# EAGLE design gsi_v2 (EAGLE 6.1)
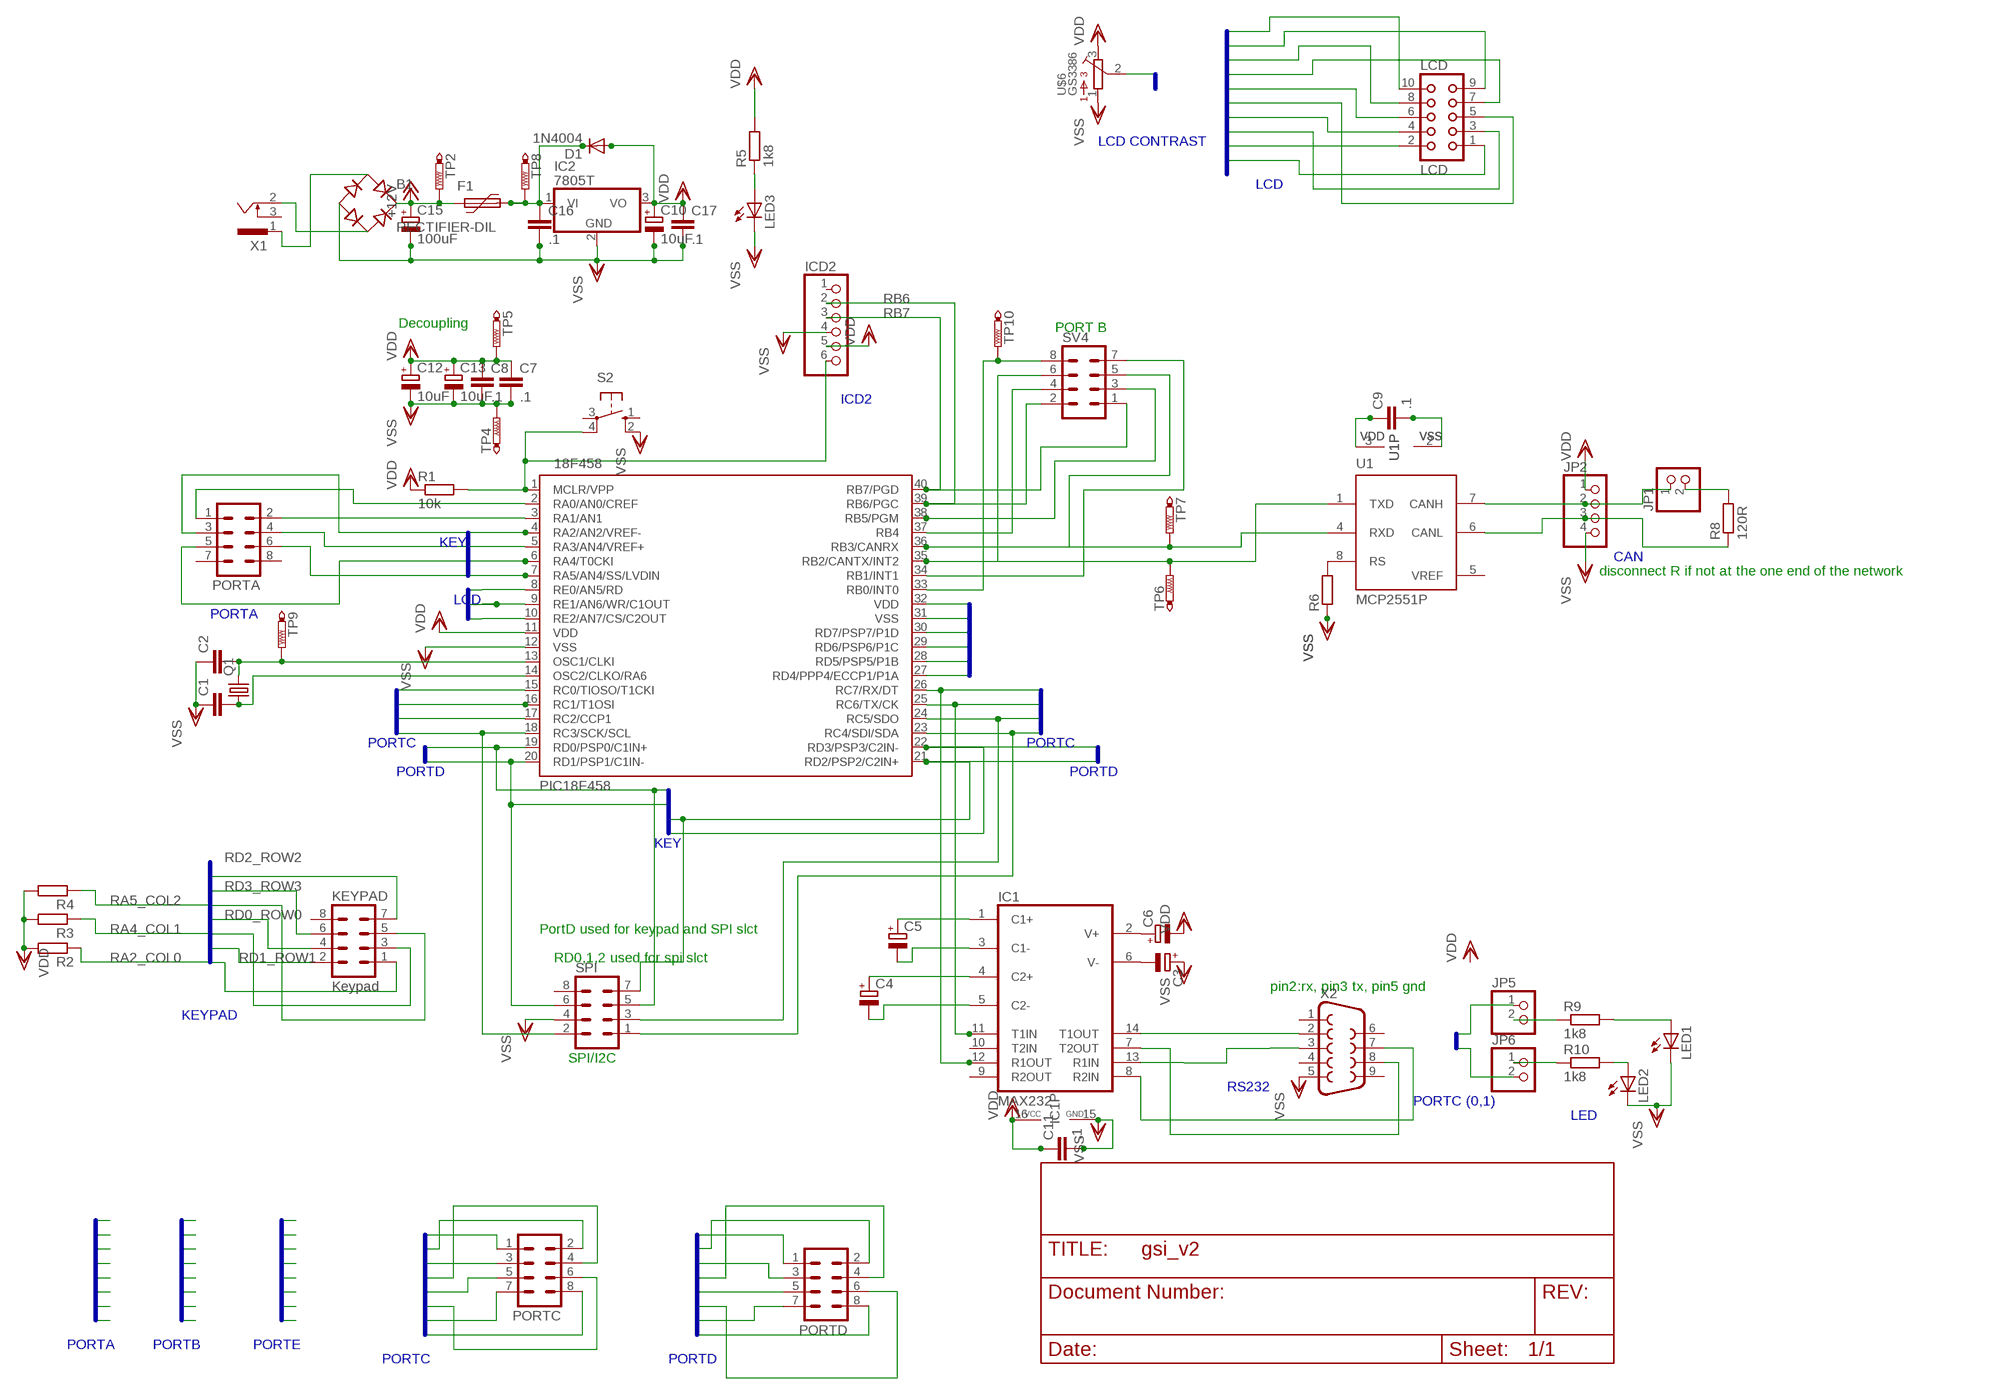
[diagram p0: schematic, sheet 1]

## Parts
B1  RECTIFIER-DIL  [B-DIL]
C1  C-EUC0603  [C0603]
C2  C-EUC0603  [C0603]
C3  CPOL-EUE2.5-6  [E2,5-6]
C4  CPOL-EUE2.5-6  [E2,5-6]
C5  CPOL-EUE2.5-6  [E2,5-6]
C6  CPOL-EUE2.5-6  [E2,5-6]
C7  .1  C-EUC0603  [C0603]
C8  .1  C-EUC0603  [C0603]
C9  .1  C-EUC0603  [C0603]
C10  10uF  CPOL-EUE2.5-5  [E2,5-5]
C11  .1  C-EUC0603  [C0603]
C12  10uF  CPOL-EUE2.5-5  [E2,5-5]
C13  10uF  CPOL-EUE2.5-5  [E2,5-5]
C15  100uF  CPOL-EUE2.5-7  [E2,5-7]
C16  .1  C-EUC0603  [C0603]
C17  .1  C-EUC0603  [C0603]
D1  1N4004  [DO41-10]
F1  MF-R055-5,1  [MF-5,1]
IC1  MAX232  [DIL16]
IC2  7805T  [TO220H]
ICD2  PINHD-1X6  [1X06]
JP1  PINHD-1X2  [1X02]
JP2  PINHD-1X4  [1X04]
JP5  PINHD-1X2  [1X02]
JP6  PINHD-1X2  [1X02]
KEYPAD  Keypad  MA04-2  [MA04-2]
LCD  LCD  CON10  [CON10]
LED1  LED5MM  [LED5MM]
LED2  LED5MM  [LED5MM]
LED3  LEDCHIPLED_1206  [CHIPLED_1206]
PORTA  MA04-2  [MA04-2]
PORTC  MA04-2  [MA04-2]
PORTD  MA04-2  [MA04-2]
Q1  CRYSTALHC18U-V  [HC18U-V]
R1  10k  R-EU_R0603  [R0603]
R2  R-EU_R0603  [R0603]
R3  R-EU_R0603  [R0603]
R4  R-EU_R0603  [R0603]
R5  1k8  R-EU_R0603  [R0603]
R6  R-EU_R0603  [R0603]
R8  120R  R-EU_0204/2V  [0204V]
R9  1k8  R-EU_R0603  [R0603]
R10  1k8  R-EU_R0603  [R0603]
S2  10-XX  [B3F-10XX]
SPI  MA04-2  [MA04-2]
SV4  MA04-2  [MA04-2]
TP2  PTR1PAD1-17  [P1-17]
TP4  PTR1PAD1-17  [P1-17]
TP5  PTR1PAD1-17  [P1-17]
TP6  PTR1PAD1-17  [P1-17]
TP7  PTR1PAD1-17  [P1-17]
TP8  PTR1PAD1-17  [P1-17]
TP9  PTR1PAD1-17  [P1-17]
TP10  PTR1PAD1-17  [P1-17]
U1  MCP2551P  [DIL8]
U$1  PIC18F458  [DIL40]
U$6  GS3386  [GS3386W]
X1  SCD-014A  [SCD-014-A]
X2  F09HP  [F09HP]

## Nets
+12V [power]: B1.+ C15.+ F1.1 TP2.1(TP)
C1+: C5.+ IC1.1(C1+)
C1-: C5.- IC1.3(C1-)
C2+: C4.+ IC1.4(C2+)
C2-: C4.- IC1.5(C2-)
CAN [power]: JP2.4 ; supply symbol labelled VSS
CANH: JP1.1 JP2.2 U1.7(CANH)
CANL: JP2.3 R8.1 U1.6(CANL)
CTS: IC1.7(T2OUT) X2.8
D4: LCD.10 U$1.27(RD4/PPP4/ECCP1/P1A)
D5: LCD.9 U$1.28(RD5/PSP5/P1B)
D6: LCD.8 U$1.29(RD6/PSP6/P1C)
D7: LCD.7 U$1.30(RD7/PSP7/P1D)
EN: LCD.1 U$1.8(RE0/AN5/RD)
LED1: LED1.A R9.2
LED2: LED2.A R10.2
MCLR: ICD2.6 R1.2 S2.4(P1) U$1.1(MCLR/VPP)
N$2: C2.2 Q1.2 TP9.1(TP) U$1.13(OSC1/CLKI)
N$3 [power]: B1.AC2 X1.2
N$4: C3.- IC1.6(V-)
N$5: C6.+ IC1.2(V+)
N$6: C1.2 Q1.1 U$1.14(OSC2/CLKO/RA6)
N$8: R6.2 U1.8(RS)
N$9 [power]: B1.AC1 X1.1
N$10 [power]: C16.1 D1.C F1.2 IC2.1(VI) TP8.1(TP)
N$13: JP6.1 R10.1
N$16: JP1.2 R8.2
N$17: JP5.2 R9.1
N$18: LED3.A R5.1
RA0: PORTA.1 U$1.2(RA0/AN0/CREF)
RA1: PORTA.2 U$1.3(RA1/AN1)
RA2_COL0: KEYPAD.1 PORTA.3 R2.1 U$1.4(RA2/AN2/VREF-)
RA3: PORTA.4 U$1.5(RA3/AN4/VREF+)
RA4_COL1: KEYPAD.3 PORTA.5 R3.1 U$1.6(RA4/T0CKI)
RA5_COL2: KEYPAD.5 PORTA.6 R4.1 U$1.7(RA5/AN4/SS/LVDIN)
RB0: SV4.8 TP10.1(TP) U$1.33(RB0/INT0)
RB1: SV4.7 U$1.34(RB1/INT1)
RB2: SV4.6 TP6.1(TP) U1.1(TXD) U$1.35(RB2/CANTX/INT2)
RB3: SV4.5 TP7.1(TP) U1.4(RXD) U$1.36(RB3/CANRX)
RB4: SV4.4 U$1.37(RB4)
RB5: SV4.3 U$1.38(RB5/PGM)
RB6: ICD2.2 SV4.2 U$1.39(RB6/PGC)
RB7: ICD2.3 SV4.1 U$1.40(RB7/PGD)
RC0: JP5.1 PORTC.1 U$1.15(RC0/TIOSO/T1CKI)
RC1: JP6.2 PORTC.2 U$1.16(RC1/T1OSI)
RC2: PORTC.3 U$1.17(RC2/CCP1)
RC3: PORTC.4 SPI.2 U$1.18(RC3/SCK/SCL)
RC4: PORTC.5 SPI.1 U$1.23(RC4/SDI/SDA)
RC5: PORTC.6 SPI.3 U$1.24(RC5/SDO)
RC6: IC1.11(T1IN) PORTC.7 U$1.25(RC6/TX/CK)
RC7: IC1.12(R1OUT) PORTC.8 U$1.26(RC7/RX/DT)
RD0_ROW0: KEYPAD.4 PORTD.1 SPI.5 U$1.19(RD0/PSP0/C1IN+)
RD1_ROW1: KEYPAD.2 PORTD.2 SPI.6 U$1.20(RD1/PSP1/C1IN-)
RD2_ROW2: KEYPAD.7 PORTD.3 SPI.7 U$1.21(RD2/PSP2/C2IN+)
RD3_ROW3: KEYPAD.6 PORTD.4 U$1.22(RD3/PSP3/C2IN-)
RD4: PORTD.5
RD5: PORTD.6
RD6: PORTD.7
RD7: PORTD.8
RS: LCD.3 U$1.10(RE2/AN7/CS/C2OUT)
RTS: IC1.8(R2IN) X2.7
RW: LCD.2 U$1.9(RE1/AN6/WR/C1OUT)
RX_232: IC1.13(R1IN) X2.3
TX_232: IC1.14(T1OUT) X2.2
VDD [power]: C6.- C7.1 C8.1 C9.1 C10.+ C11.1 C12.+ C13.+ C17.1 D1.A IC1.16(VCC) IC2.3(VO) ICD2.5 JP2.1 LCD.4 R1.1 R2.2 R3.2 R4.2 R5.2 TP5.1(TP) U1.3(VDD) U$1.11(VDD) U$1.32(VDD) U$6.3
VO: LCD.6 U$6.2
VSS [power]: B1.- C1.1 C2.1 C3.+ C7.2 C8.2 C9.2 C10.- C11.2 C12.- C13.- C15.- C16.2 C17.2 IC1.15(GND) IC2.2(GND) ICD2.4 LCD.5 LED1.K(C) LED2.K(C) LED3.C R6.1 S2.2(S1) SPI.4 TP4.1(TP) U1.2(VSS) U$1.12(VSS) U$1.31(VSS) U$6.1 X2.5
Unconnected: IC1.9(R2OUT) IC1.10(T2IN) ICD2.1 KEYPAD.8 PORTA.7 PORTA.8 S2.1(S) S2.3(P) SPI.8 X1.3 X2.1 X2.4 X2.6 X2.9

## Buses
LCD_BUS
KEYPAD_BUS
PORTD
PORTC
PORTE
PORTB
PORTA
VDD,VSS,RS,VO,EN,RW,D4,D5,D6,D7

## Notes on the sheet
- LCD CONTRAST
- LCD
- Decoupling
- PORT B
- ICD2
- KEY
- CAN
- disconnect R if not at the one end of the network
- LCD
- PORTA
- PORTC | PORTC
- PORTD | PORTD
- KEY
- PortD used for keypad and SPI slct
- RD0,1,2 used for spi slct
- pin2:rx, pin3 tx, pin5 gnd
- KEYPAD
- SPI/I2C
- RS232
- PORTC (0,1)
- LED
- PORTA | PORTB | PORTE
- PORTC | PORTD

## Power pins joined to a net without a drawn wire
VREF: U1.5(VREF)

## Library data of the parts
B1 = rectifier:RECTIFIER-: Rectifier
C1 C2 C7-C9 C11 C16 C17 = rcl:C-EU: CAPACITOR, European symbol
C3-C6 C10 C12 C13 C15 = rcl:CPOL-EU: POLARIZED CAPACITOR, European symbol
D1 = diode:1N4004: DIODE
F1 = bourns:MF-R055: MultiFuse
IC1 = maxim:MAX232: RS232 TRANSEIVER
IC2 = linear:78*: Positive VOLTAGE REGULATOR Source: http://cache.national.com/ds/LM/LM78L05.pdf http://www.fairchildsemi.com/ds/LM/LM7805.pdf
ICD2 = pinhead:PINHD-1X6: PIN HEADER
JP1 JP5 JP6 = pinhead:PINHD-1X2: PIN HEADER
JP2 = pinhead:PINHD-1X4: PIN HEADER
KEYPAD PORTA PORTC PORTD SPI SV4 = con-lstb:MA04-2: PIN HEADER
LCD = con-harting:CON10: CONNECTOR; OC_FARNELL: unknown; OC_NEWARK: unknown
LED1-LED3 = led:LED: LED
Q1 = crystal:CRYSTAL: CRYSTAL
R1-R6 R8-R10 = rcl:R-EU_: RESISTOR, European symbol
S2 = switch-omron:10-XX: OMRON SWITCH
TP2 TP4-TP10 = testpad:PTR1: TEST PIN
U1 = microchip_can:MCP2551: High Speed CAN tranceiver
U$1 = gs:PIC18F458
U$6 = gs:GS3386: GS larger pads
X1 = con-shiua-chyuan:SCD-014A: Power Jack 2.5mm
X2 = con-subd:F09: SUB-D

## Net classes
0 default: width 0.457 mm, drill 0.813 mm, clearance 0.254 mm
1 power: width 1.016 mm, drill 0.813 mm, clearance 0.508 mm
2 digital: width 0.457 mm, drill 0.813 mm, clearance 0.254 mm

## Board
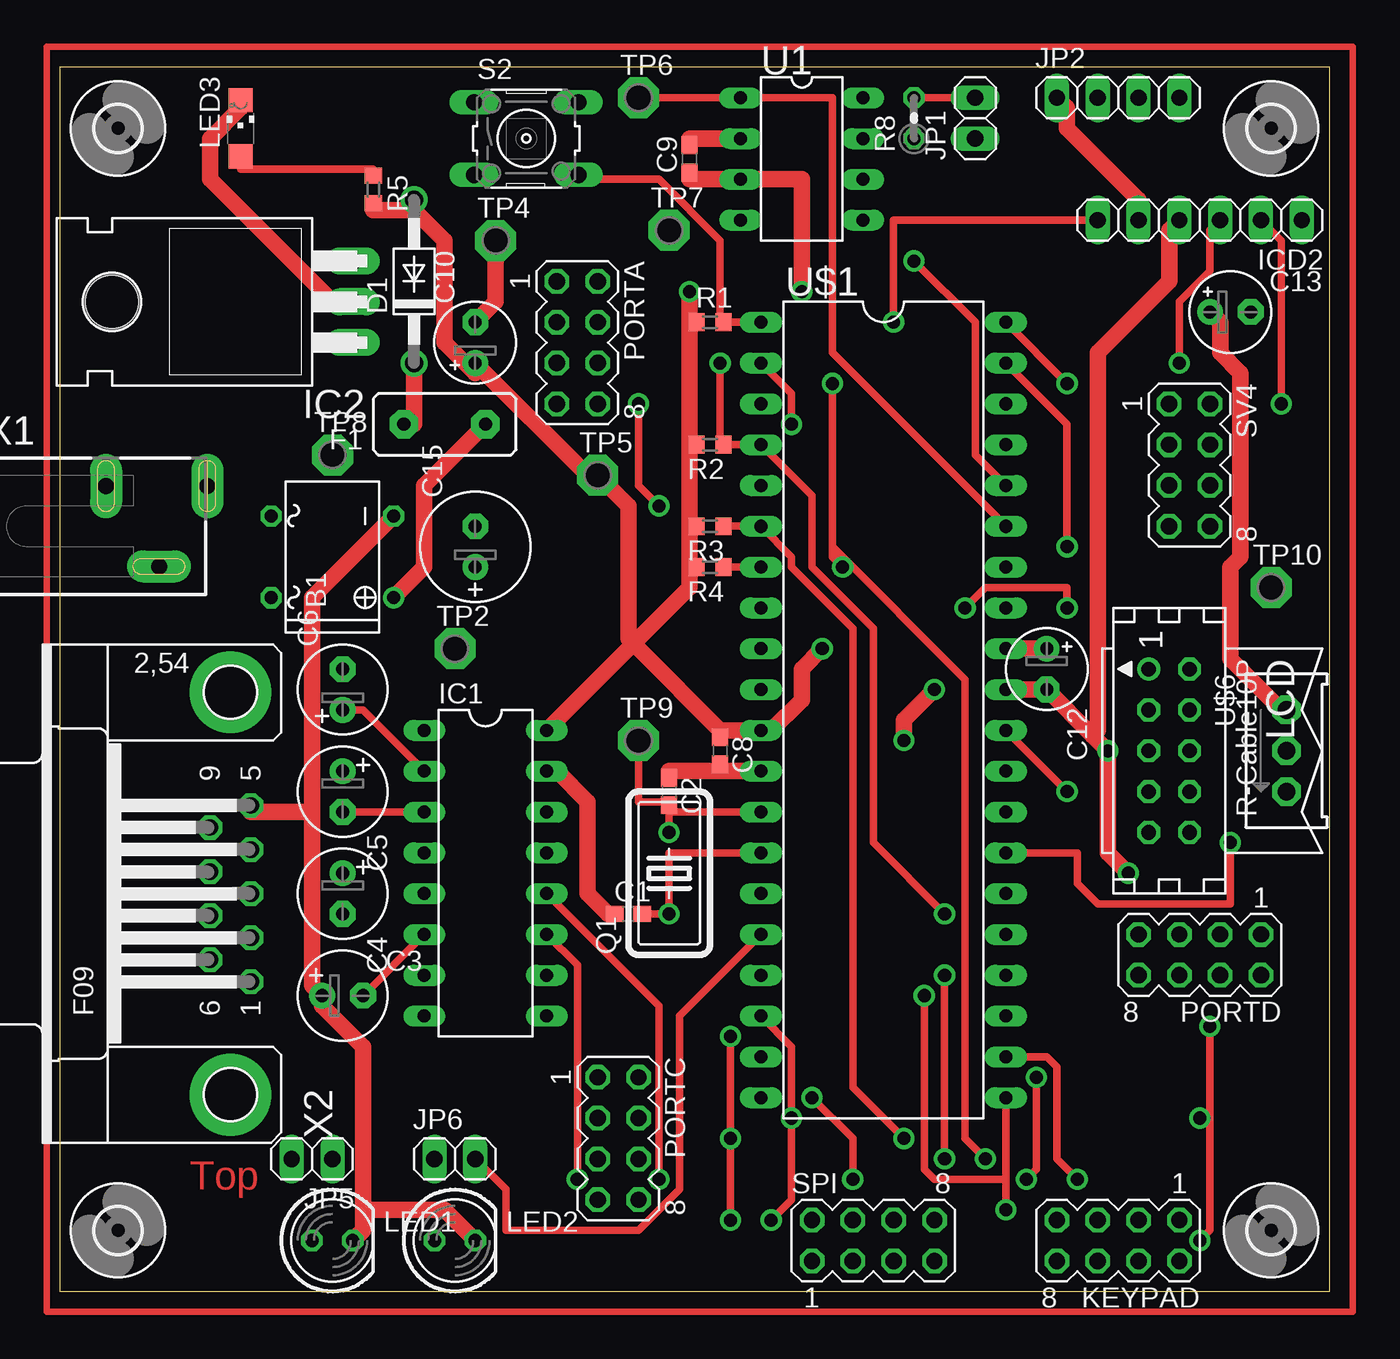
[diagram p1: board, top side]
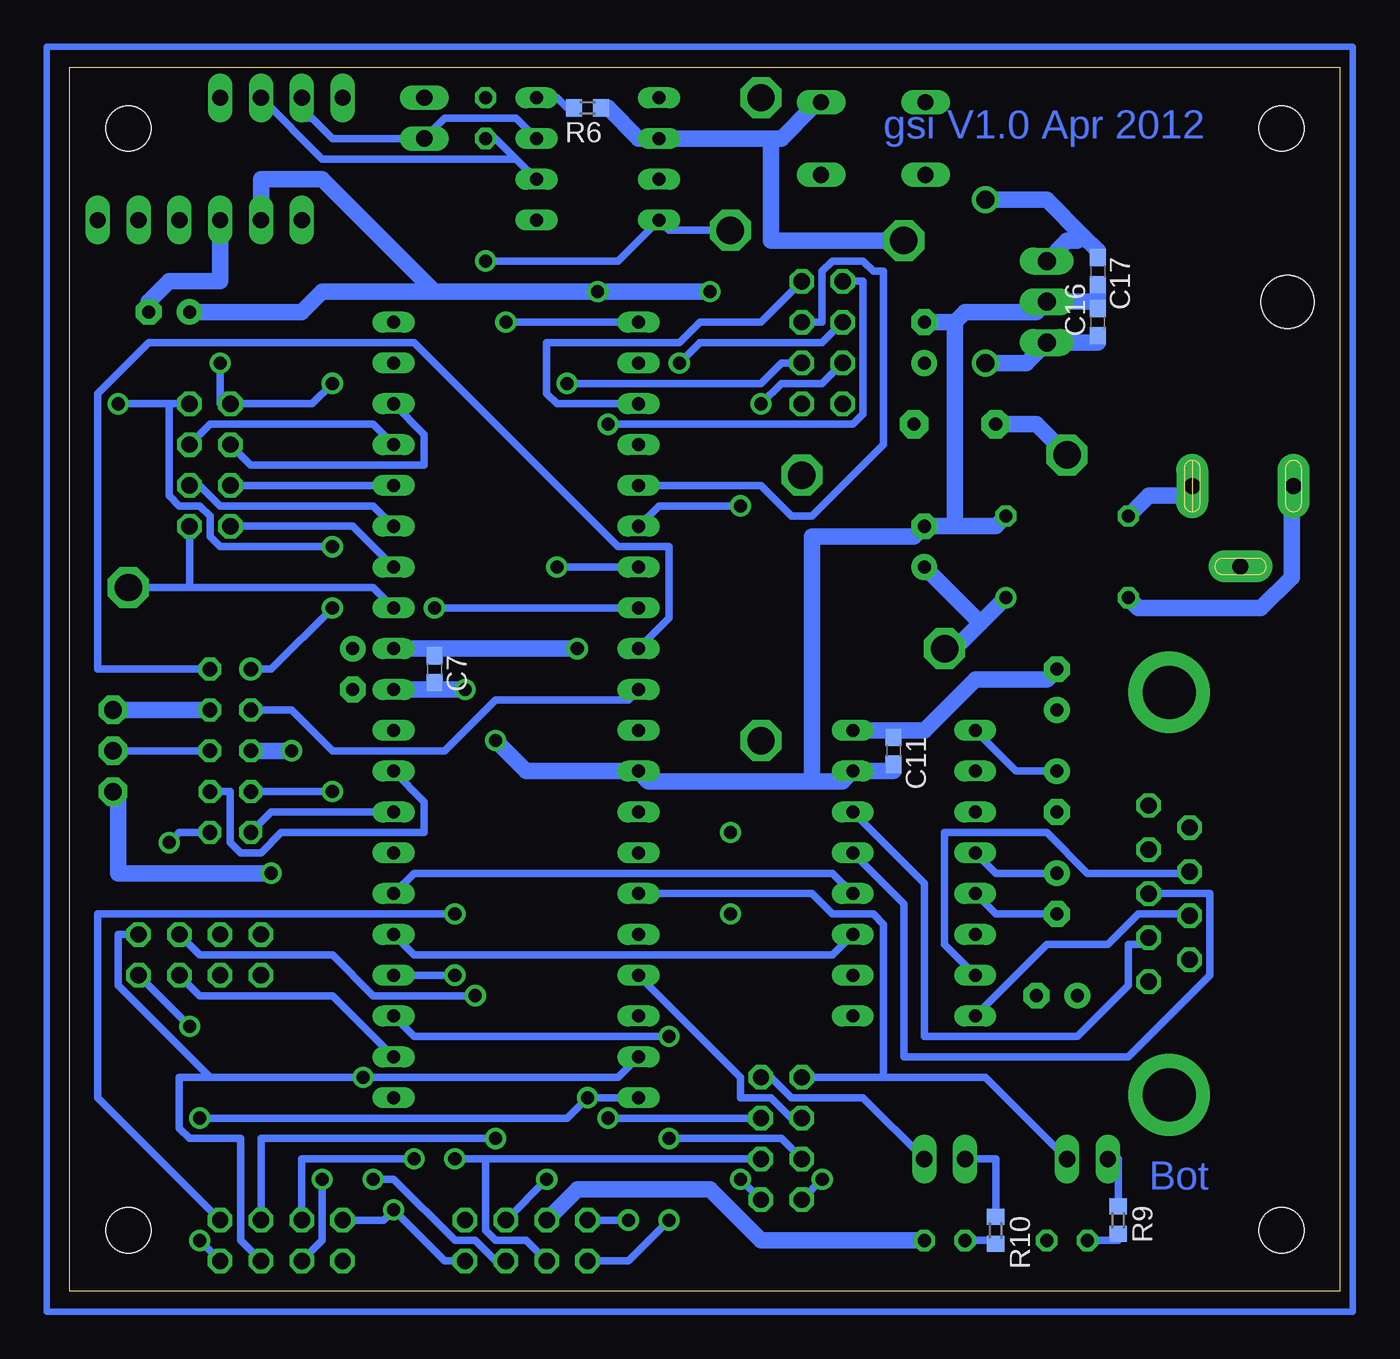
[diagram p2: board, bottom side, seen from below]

Size 79.05 x 76.19 mm. Coordinates in mm from the lower left corner, seen from the top.
Outline: 0,0 79.05,0 79.05,76.19 0,76.19 0,0
Copper layers (1*16): Top 0.035mm / dielectric 1.5mm / Bottom 0.035mm
Design rules: minimum track width 10mil, minimum drill 24mil, track to track 10mil, track to pad 10mil, pad to pad 10mil, via to via 10mil, smd to smd 10mil, copper to edge 40mil, drill to drill 10mil, minimum pad ring 10mil, minimum via ring 10mil, stop-mask expansion 4mil, vias tented up to drill 0mil, thermal gap 10mil
tRestrict: area 33.5,4.4 to 36,14.6; area 45.6,1.9 to 55.7,4.4; area 26.5,69.8 to 31.6,74.9; area 67.8,46.4 to 72.9,56.5; area 65.9,18.4 to 76,23.5; area 66.5,27.3 to 71.6,41.3; area 60.8,1.9 to 69.7,5.1; area 30.3,54.6 to 34.1,63.5

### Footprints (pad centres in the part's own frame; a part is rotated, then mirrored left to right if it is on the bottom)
B-DIL = drill 0.813: + -2.54,-3.81 | drill 0.813 octagon: - 2.54,-3.81; AC1 2.54,3.81; AC2 -2.54,3.81
C0603 = smd 1.1 x 1: 1 -0.85,0; 2 0.85,0
E2,5-6 = drill 0.813 pad 1.6: + -1.27,0 | drill 0.813 pad 1.6 octagon: - 1.27,0
E2,5-5 = drill 0.813 pad 1.6: + -1.27,0 | drill 0.813 pad 1.6 octagon: - 1.27,0
E2,5-7 = drill 0.813 pad 1.6: + -1.27,0 | drill 0.813 pad 1.6 octagon: - 1.27,0
DO41-10 = drill 1.118: A 5.08,0; C -5.08,0
MF-5,1 = drill 0.813 pad 1.778 octagon: 1 -2.54,0; 2 2.54,0
DIL16 = drill 0.813 long: 1 -8.89,-3.81; 2 -6.35,-3.81; 3 -3.81,-3.81; 4 -1.27,-3.81; 5 1.27,-3.81; 6 3.81,-3.81; 7 6.35,-3.81; 8 8.89,-3.81; 9 8.89,3.81; 10 6.35,3.81; 11 3.81,3.81; 12 1.27,3.81; 13 -1.27,3.81; 14 -3.81,3.81; 15 -6.35,3.81; 16 -8.89,3.81
TO220H = drill 1.118 long: 1 -2.54,-10.16; 2 0,-10.16; 3 2.54,-10.16 | hole 3.302: 0,4.826
1X06 = drill 1.016 long: 1 -6.35,0; 2 -3.81,0; 3 -1.27,0; 4 1.27,0; 5 3.81,0; 6 6.35,0
1X02 = drill 1.016 long: 1 -1.27,0; 2 1.27,0
1X04 = drill 1.016 long: 1 -3.81,0; 2 -1.27,0; 3 1.27,0; 4 3.81,0
MA04-2 = drill 1.016 octagon: 1 -3.81,-1.27; 2 -3.81,1.27; 3 -1.27,-1.27; 4 -1.27,1.27; 5 1.27,-1.27; 6 1.27,1.27; 7 3.81,-1.27; 8 3.81,1.27
CON10 = drill 0.914: 1 -5.08,-1.27 | drill 0.914 octagon: 2 -5.08,1.27; 3 -2.54,-1.27; 4 -2.54,1.27; 5 0,-1.27; 6 0,1.27; 7 2.54,-1.27; 8 2.54,1.27; 9 5.08,-1.27; 10 5.08,1.27
LED5MM = drill 0.813 octagon: A -1.27,0; K 1.27,0
CHIPLED_1206 = smd 1.5 x 1.5: A 0,-1.75; C 0,1.75
HC18U-V = drill 0.813: 1 -2.54,0; 2 2.54,0
R0603 = smd 1 x 1.1: 1 -0.85,0; 2 0.85,0
0204V = drill 0.813 octagon: 1 -1.27,0; 2 1.27,0
B3F-10XX = drill 1.016 long: 1 -3.251,2.261; 2 3.251,2.261; 3 -3.251,-2.261; 4 3.251,-2.261
P1-17 = drill 1.702 pad 2.54 octagon: 1 0,0
DIL8 = drill 0.813 long: 1 -3.81,-3.81; 2 -1.27,-3.81; 3 1.27,-3.81; 4 3.81,-3.81; 5 3.81,3.81; 6 1.27,3.81; 7 -1.27,3.81; 8 -3.81,3.81
DIL40 = drill 0.813 long: 1 -24.13,-7.62; 2 -21.59,-7.62; 3 -19.05,-7.62; 4 -16.51,-7.62; 5 -13.97,-7.62; 6 -11.43,-7.62; 7 -8.89,-7.62; 8 -6.35,-7.62; 9 -3.81,-7.62; 10 -1.27,-7.62; 11 1.27,-7.62; 12 3.81,-7.62; 13 6.35,-7.62; 14 8.89,-7.62; 15 11.43,-7.62; 16 13.97,-7.62; 17 16.51,-7.62; 18 19.05,-7.62; 19 21.59,-7.62; 20 24.13,-7.62; 21 24.13,7.62; 22 21.59,7.62; 23 19.05,7.62; 24 16.51,7.62; 25 13.97,7.62; 26 11.43,7.62; 27 8.89,7.62; 28 6.35,7.62; 29 3.81,7.62; 30 1.27,7.62; 31 -1.27,7.62; 32 -3.81,7.62; 33 -6.35,7.62; 34 -8.89,7.62; 35 -11.43,7.62; 36 -13.97,7.62; 37 -16.51,7.62; 38 -19.05,7.62; 39 -21.59,7.62; 40 -24.13,7.62
2,8 = hole 2.8: 0,0
GS3386W = drill 1.1 pad 1.778 octagon: 1 2.54,0.318; 2 0,0.318; 3 -2.54,0.318
SCD-014-A = drill 1 pad 2 long: 1 -2.5,13.8; 2 -2.5,7.5; 3 2.5,10.8
F09HP = drill 1.016 octagon: 1 -5.486,-1.27; 2 -2.743,-1.27; 3 0,-1.27; 4 2.743,-1.27; 5 5.486,-1.27; 6 -4.115,1.27; 7 -1.372,1.27; 8 1.372,1.27; 9 4.115,1.27 | drill 3.302 pad 5.08: G1 -12.522,0; G2 12.522,0

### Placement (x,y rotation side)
B1  16.98,45.71 90 top
C1  35.39,23.49 0 top
C2  37.94,31.11 270 top
C3  17.61,18.41 0 top
C4  17.61,24.76 270 top
C5  17.61,31.11 270 top
C6  17.61,37.46 90 top
C7  56.35,38.73 270 bottom
C8  41.11,33.65 270 top
C9  39.2,70.48 90 top
C10  25.87,59.05 90 top
C11  27.78,33.65 270 bottom
C12  61.43,38.73 270 top
C13  72.86,60.95 0 top
C15  25.87,46.35 90 top
C16  15.07,60.32 90 bottom
C17  15.07,63.5 270 bottom
D1  22.06,62.86 90 top
F1  23.96,53.97 180 top
IC1  26.5,26.03 270 top
IC2  8.09,61.59 90 top
ICD2  70.95,66.67 180 top
JP1  56.98,73.02 90 top
JP2  65.88,74.29 0 top
JP5  15.71,8.25 180 top
JP6  24.6,8.25 0 top
KEYPAD  65.88,3.17 180 top
LCD  69.05,33.65 270 top
LED1  16.98,3.17 0 top
LED2  24.6,3.17 0 top
LED3  11.26,72.39 0 top
PORTA  32.22,59.05 270 top
PORTC  34.76,9.52 270 top
PORTD  70.95,20.95 180 top
Q1  37.94,26.03 90 top
R1  40.47,60.32 0 top
R2  40.47,52.7 180 top
R3  40.47,47.62 180 top
R4  40.47,45.08 180 top
R5  19.52,68.58 270 top
R6  46.82,73.66 180 bottom
R8  53.17,73.02 90 top
R9  13.8,4.44 270 bottom
R10  21.43,3.8 270 bottom
S2  29.04,71.75 0 top
SPI  50.63,3.17 0 top
SV4  70.32,51.43 270 top
TP2  24.6,40 0 top
TP4  27.14,65.4 0 top
TP5  33.49,50.8 0 top
TP6  36.03,74.29 0 top
TP7  37.94,66.03 0 top
TP8  16.98,52.06 0 top
TP9  36.03,34.28 0 top
TP10  75.4,43.81 0 top
U1  46.19,70.48 270 top
U$1  51.27,36.19 270 top
U$2  [2,8]  3.64,72.39 0 top
U$3  [2,8]  75.4,72.39 0 top
U$4  [2,8]  75.4,3.8 0 top
U$5  [2,8]  3.64,3.8 0 top
U$6  76.03,33.65 270 top
X1  -4.61,47.62 270 top
X2  10.63,24.76 90 top

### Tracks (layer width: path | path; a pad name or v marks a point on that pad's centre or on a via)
+12V
  Top 1.016: F1.1 22.69,50.16 22.69,45.08 B1.+
  Bottom 1.016: 22.38,41.59 23.96,40 TP2.1 | 22.38,41.59 B1.+ | C15.+ 22.69,41.91 22.38,41.59
C1+
  Bottom 0.457: IC1.1 20.15,32.38 C5.+
C1-
  Top 0.457: C5.- IC1.3
C2+
  Bottom 0.457: IC1.4 21.43,26.03 C4.+
C2-
  Bottom 0.457: IC1.5 21.43,23.49 C4.-
CANH
  Bottom 0.457: U1.7 51.27,73.02 55.71,73.02 JP1.1 62.7,71.75 63.97,73.02 64.6,73.02 JP2.2
CANL
  Bottom 0.457: 51.27,70.48 52.54,71.75 R8.1 | 51.27,70.48 U1.6 | JP2.3 63.33,70.48 51.27,70.48
CTS
  Bottom 0.457: IC1.7 24.6,21.59 24.6,28.57 18.25,28.57 15.71,26.03 9.36,26.03 X2.8
D4  (via drill 0.81)
  Top 0.457: U$1.27 63.33,27.3 63.33,25.4 64.6,24.12 72.86,24.12 v72.86,27.94
  Bottom 0.457: v72.86,27.94 72.22,28.57 LCD.10
D5
  Bottom 0.457: U$1.28 66.51,29.84 LCD.9
D6
  Bottom 0.457: U$1.29 56.98,30.48 56.98,28.57 65.88,28.57 67.14,27.3 68.41,27.3 69.05,27.94 69.05,31.11 LCD.8
D7  (via drill 0.81)
  Top 0.457: v62.7,31.11 U$1.30
  Bottom 0.457: LCD.7 v62.7,31.11
EN  (via drill 0.81)
  Top 0.457: v56.35,42.54 57.62,43.81 62.7,43.81 v62.7,42.54
  Bottom 0.457: v56.35,42.54 U$1.8 | v62.7,42.54 66.51,38.73 LCD.1
LED1
  Bottom 0.457: LED1.A 13.8,3.17 R9.2
LED2
  Bottom 0.457: LED2.A 21.43,3.17 R10.2
MCLR  (via drill 0.81)
  Top 0.457: U$1.1 41.75,60.32 R1.2 41.11,60.32 41.11,65.4 37.3,69.21 32.86,69.21 S2.4 | ICD2.6 51.91,66.67 v51.91,60.32
  Bottom 0.457: U$1.1 v51.91,60.32
N$1
  Top 0.406: -0.8,77.47 -0.8,-1.27 80.48,-1.27 80.48,77.47 -0.8,77.47
N$2
  Top 0.457: Q1.2 37.94,29.84 | 37.94,29.84 C2.2 | 37.94,29.84 U$1.13 | 37.94,29.84 C2.2 | TP9.1 36.03,30.48 37.94,30.48 C2.2
N$3
  Bottom 1.016: B1.AC2 12.54,42.54 4.91,42.54 3.01,44.45 3.01,49.52 X1.2
N$4
  Top 0.457: C3.- IC1.6
N$5
  Top 0.457: IC1.2 18.89,36.19 C6.+
N$6
  Top 0.457: C1.2 36.66,23.49 Q1.1 37.94,27.3 U$1.14
N$7
  Bottom 0.406: -0.8,77.47 80.48,77.47 80.48,-1.27 -0.8,-1.27 -0.8,77.47
N$8
  Bottom 0.457: U1.8 48.73,74.29 48.09,73.66 R6.2
N$9
  Bottom 1.016: B1.AC1 11.9,49.52 9.36,49.52 X1.1
N$10
  Top 1.016: D1.C 22.06,53.97 F1.2
  Bottom 1.016: C16.1 15.07,59.05 IC2.1 19.52,57.78 D1.C | TP8.1 18.89,53.97 F1.2 | F1.2
N$11  (via drill 0.6 pad 2.54)
  other vias: 3.64,72.39
N$12  (via drill 0.6 pad 2.54)
  other vias: 75.4,72.39
N$13
  Bottom 0.457: JP6.1 21.43,8.25 21.43,5.08 R10.1
N$14  (via drill 0.6 pad 2.54)
  other vias: 3.64,3.8
N$15  (via drill 0.6 pad 2.54)
  other vias: 75.4,3.8
N$16
  Top 0.457: JP1.2 R8.2
N$17
  Bottom 0.457: JP5.2 13.8,8.25 13.8,5.71 R9.1
N$18
  Top 0.457: R5.1 19.52,69.84 11.26,69.84 11.26,70.48 LED3.A
RA0  (via drill 0.81)
  Top 0.457: U$1.2 45.55,55.88 v45.55,53.97
  Bottom 0.457: v45.55,53.97 30.32,53.97 29.68,54.6 29.68,62.86 PORTA.1
RA1
  Bottom 0.457: U$1.3 48.73,55.24 49.36,55.88 49.36,59.05 41.11,59.05 39.84,60.32 36.03,60.32 PORTA.2
RA2_COL0  (via drill 0.81)
  Top 0.457: v41.11,57.78 41.11,52.7 R2.1 41.75,52.7 U$1.4 46.82,49.52 46.82,45.08 50.63,41.27 50.63,27.94 v55.08,23.49
  Bottom 0.457: v41.11,57.78 39.84,59.05 32.22,59.05 PORTA.3 | KEYPAD.1 77.3,12.06 77.3,23.49 v55.08,23.49
RA3
  Bottom 0.457: U$1.5 36.03,50.16 34.12,48.25 32.86,48.25 28.41,52.7 28.41,63.5 29.04,63.5 29.68,64.13 31.58,64.13 32.22,63.5 32.22,60.32 PORTA.4
RA4_COL1  (via drill 0.81)
  Top 0.457: R3.1 41.75,47.62 U$1.6 45.55,45.71 45.55,45.08 49.36,41.27 49.36,12.7 v52.54,9.52 | v37.3,48.89 36.03,50.16 v36.03,55.24
  Bottom 0.457: U$1.6 42.38,48.89 v37.3,48.89 | v36.03,55.24 34.76,56.51 32.22,56.51 PORTA.5 | KEYPAD.3 67.14,9.52 v52.54,9.52
RA5_COL2  (via drill 0.81)
  Top 0.457: U$1.7 41.75,45.08 R4.1 | v48.73,45.08 48.09,45.71 48.09,46.35 | v48.09,56.51 48.09,46.35 | v57.62,8.25 56.35,9.52 56.35,38.09 48.09,46.35
  Bottom 0.457: v48.73,45.08 U$1.7 | v48.09,56.51 36.03,56.51 34.76,57.78 PORTA.6 | KEYPAD.5 64.6,8.25 v57.62,8.25
RB0
  Bottom 0.457: U$1.33 60.16,43.81 71.59,43.81 | TP10.1 71.59,43.81 | 71.59,43.81 SV4.8
RB1
  Bottom 0.457: U$1.34 61.43,47.62 SV4.7
RB2
  Top 0.457: TP6.1 U1.1 48.09,74.29 48.09,58.41 U$1.35
  Bottom 0.457: U$1.35 60.16,48.89 69.69,48.89 70.95,50.16 SV4.6
RB3  (via drill 0.81)
  Top 0.457: v53.17,64.13 56.98,60.32 56.98,52.06 U$1.36
  Bottom 0.457: TP7.1 41.75,66.03 U1.4 44.92,64.13 v53.17,64.13 | SV4.5 U$1.36
RB4
  Bottom 0.457: U$1.37 60.16,53.97 70.32,53.97 SV4.4
RB5
  Bottom 0.457: U$1.38 56.98,53.34 56.98,51.43 67.78,51.43 SV4.3
RB6  (via drill 0.81)
  Top 0.457: U$1.39 62.7,53.97 v62.7,46.35 | ICD2.2 76.03,65.4 v76.03,55.24
  Bottom 0.457: v62.7,46.35 69.69,46.35 70.32,46.98 70.32,48.25 70.95,48.89 72.22,48.89 72.86,49.52 72.86,55.24 | SV4.2 72.86,55.24 | 72.86,55.24 v76.03,55.24
RB7  (via drill 0.81)
  Top 0.457: v62.7,56.51 U$1.40 | ICD2.3 71.59,66.03 71.59,63.5 69.69,61.59 v69.69,57.78
  Bottom 0.457: v62.7,56.51 63.97,55.24 SV4.1 69.69,55.24 v69.69,57.78
RC0
  Bottom 0.457: U$1.15 32.86,24.76 31.58,23.49 29.04,23.49 28.41,22.85 28.41,13.33 | PORTC.1 28.41,13.33 | JP5.1 22.06,13.33 28.41,13.33
RC1
  Top 0.457: U$1.16 38.57,17.14 38.57,6.35 36.03,3.8 27.78,3.8 27.78,6.35 JP6.2
  Bottom 0.457: PORTC.2 35.39,13.33 34.12,12.06 29.68,12.06 JP6.2
RC2
  Bottom 0.457: U$1.17 37.3,13.33 37.3,12.06 35.39,12.06 34.12,10.79 PORTC.3
RC3  (via drill 0.81)
  Top 0.457: U$1.18 45.55,15.24 v45.55,10.79 45.55,5.71 v44.28,4.44
  Bottom 0.457: PORTC.4 v45.55,10.79 | v44.28,4.44 SPI.2
RC4  (via drill 0.81)
  Top 0.457: v41.75,4.44 v41.75,9.52 v41.75,15.87
  Bottom 0.457: U$1.23 57.62,15.87 v41.75,15.87 | v41.75,4.44 44.28,1.9 SPI.1 | PORTC.5 34.76,9.52 v41.75,9.52
RC5  (via drill 0.81)
  Top 0.457: v55.08,8.25 v55.08,19.68
  Bottom 0.457: v55.08,19.68 U$1.24 | PORTC.6 53.17,8.25 | 53.17,8.25 v55.08,8.25 | SPI.3 50.63,3.17 52.54,3.17 53.17,3.8 53.17,8.25
RC6  (via drill 0.81)
  Top 0.457: v32.22,6.98 32.22,20.31 IC1.11
  Bottom 0.457: IC1.11 31.58,20.95 57.62,20.95 U$1.25 | v32.22,6.98 PORTC.7
RC7  (via drill 0.81)
  Top 0.457: v37.3,6.98 37.3,17.77 IC1.12
  Bottom 0.457: IC1.12 31.58,26.03 57.62,26.03 U$1.26 | v37.3,6.98 PORTC.8
RD0_ROW0  (via drill 0.81)
  Top 0.457: v60.16,6.98 60.8,7.62 v60.8,13.33
  Bottom 0.457: U$1.19 44.92,13.33 v60.8,13.33 70.32,13.33 | 70.32,13.33 76.03,19.05 76.03,22.22 PORTD.1 | SPI.5 52.54,1.9 53.81,3.17 55.08,3.17 58.89,6.98 v60.16,6.98 | KEYPAD.4 68.41,3.17 68.41,9.52 71.59,9.52 72.22,10.15 72.22,13.33 70.32,13.33
RD1_ROW1  (via drill 0.81)
  Top 0.457: v46.82,12.06 49.36,9.52 v49.36,6.98 | v70.95,3.17 71.59,3.8 71.59,10.79 | v71.59,16.51 71.59,10.79 | 71.59,10.79 v70.95,10.79
  Bottom 0.457: U$1.20 v46.82,12.06 48.09,10.79 v70.95,10.79 | SPI.6 v49.36,6.98 | v70.95,3.17 KEYPAD.2 | PORTD.2 v71.59,16.51
RD2_ROW2  (via drill 0.81)
  Top 0.457: v58.89,5.08 58.89,6.98 | 58.89,6.98 U$1.21 | v53.81,18.41 53.81,7.62 54.44,6.98 58.89,6.98
  Bottom 0.457: KEYPAD.7 59.52,4.44 v58.89,5.08 55.71,1.9 SPI.7 | PORTD.3 70.95,20.95 62.7,20.95 60.16,18.41 v53.81,18.41
RD3_ROW3  (via drill 0.81)
  Top 0.457: v63.33,6.98 62.06,8.25 62.06,13.97 61.43,14.6 U$1.22
  Bottom 0.457: U$1.22 62.7,18.41 70.95,18.41 PORTD.4 | KEYPAD.6 63.33,3.17 v63.33,6.98
RS
  Bottom 0.457: U$1.10 44.28,36.82 52.54,36.82 55.71,33.65 62.7,33.65 65.24,36.19 LCD.3
RTS
  Bottom 0.457: IC1.8 18.25,21.59 14.44,21.59 12.54,23.49 9.36,23.49 X2.7
RW
  Bottom 0.457: U$1.9 41.75,41.91 41.75,46.35 44.92,46.35 57.62,59.05 74.13,59.05 77.3,55.88 77.3,38.73 LCD.2
RX_232
  Bottom 0.457: IC1.13 27.14,24.12 27.14,14.6 13.17,14.6 8.09,19.68 8.09,24.76 X2.3
TX_232
  Bottom 0.457: IC1.14 25.87,25.4 25.87,15.87 16.35,15.87 13.17,19.05 13.17,21.59 11.9,21.59 X2.2
VDD  (via drill 0.81)
  Top 1.016: JP2.1 62.7,73.66 62.7,72.39 67.14,67.94 ICD2.5 | C9.1 39.2,69.21 U1.3 46.19,69.21 v46.19,62.22 | C13.+ 72.22,60.32 72.22,58.41 73.49,57.14 73.49,45.71 72.86,45.08 72.86,39.36 76.03,36.19 U$6.3 | 22.06,67.3 19.52,67.3 R5.2 | 22.06,67.3 D1.A 22.06,67.3 | 22.06,67.3 23.96,65.4 23.96,59.05 25.87,57.14 C10.+ 32.86,50.8 TP5.1 35.39,48.89 35.39,40.63 35.71,40.32 | C12.+ U$1.32 | 41.11,34.92 U$1.11 44.28,34.92 46.19,36.82 46.19,38.73 v47.46,40 | 41.11,34.92 C8.1 41.11,34.92 | 39.2,47.62 39.2,45.08 | 39.2,45.08 R4.2 39.2,45.08 | 39.2,47.62 R3.2 39.2,47.62 | 39.2,47.62 39.2,52.7 | 39.2,52.7 R2.2 39.2,52.7 | 39.2,52.7 39.2,60.32 | 39.2,60.32 R1.1 39.2,60.32 | 35.71,40.32 39.2,43.81 39.2,45.08 | 35.71,40.32 IC1.16 | 41.11,34.92 36.03,40 35.71,40.32 | 39.2,60.32 v39.2,62.22
  Bottom 1.016: LCD.4 76.03,36.19 U$6.3 | 56.35,62.22 63.33,62.22 64.6,60.95 C13.+ | 56.35,62.22 v46.19,62.22 v39.2,62.22 | ICD2.5 67.14,69.21 63.33,69.21 56.35,62.22 | 16.03,65.72 18.25,67.94 D1.A | 16.03,65.72 15.07,64.77 C17.1 | IC2.3 16.98,65.4 16.35,65.4 16.03,65.72 | U$1.32 56.35,40 | 56.35,40 C7.1 56.35,40 | IC1.16 27.78,34.92 | 27.78,34.92 C11.1 27.78,34.92 | C6.- 18.25,38.09 22.69,38.09 25.87,34.92 27.78,34.92 | v47.46,40 56.35,40
VO
  Bottom 0.457: LCD.6 76.03,33.65 U$6.2
VSS  (via drill 0.81)
  Top 1.016: LED1.K 18.89,3.8 18.89,5.08 | 18.89,5.08 18.89,15.24 16.35,17.77 C3.+ 15.71,19.05 15.71,29.84 | LED2.K 23.96,5.08 18.89,5.08 | 15.71,29.84 11.9,29.84 X2.5 | 64.29,34.6 C12.- U$1.31 | 64.29,34.6 v65.24,33.65 65.24,27.3 v66.51,26.03 | ICD2.4 69.05,66.03 69.05,62.86 64.6,58.41 64.6,34.92 64.29,34.6 | 41.11,32.38 37.94,32.38 C2.1 | 41.11,32.38 C8.2 41.11,32.38 | U$1.12 41.11,32.38 | IC1.15 30.95,32.38 32.86,30.48 32.86,24.76 34.12,23.49 C1.1 | IC2.2 16.98,61.59 9.36,69.21 9.36,71.75 11.26,73.66 LED3.C | U1.2 39.2,71.75 C9.2 | C10.- 27.14,61.59 TP4.1 | v54.44,37.46 52.54,35.55 v52.54,34.28 | 15.71,29.84 15.71,43.17 B1.-
  Bottom 1.016: SPI.4 47.46,6.35 39.2,6.35 36.03,3.17 LED2.K | ICD2.4 69.69,62.86 72.86,62.86 74.13,61.59 C13.- | U$1.31 56.35,37.46 | 56.35,37.46 C7.2 56.35,37.46 | v65.24,33.65 LCD.5 | v66.51,26.03 76.03,26.03 76.03,31.11 U$6.1 | C11.2 27.78,32.38 IC1.15 30.95,31.74 32.86,31.74 | 32.86,31.74 43.02,31.74 U$1.12 50.63,32.38 v52.54,34.28 | 15.07,61.59 15.07,62.22 C17.2 | 15.07,61.59 C16.2 15.07,61.59 | 15.07,61.59 IC2.2 18.89,60.95 23.33,60.95 23.96,60.32 | R6.1 45.55,73.66 43.65,71.75 U1.2 35.39,71.75 | 35.39,71.75 34.76,71.75 32.86,73.66 S2.2 | B1.- 21.43,47.62 23.96,47.62 | 23.96,47.62 C15.- 26.5,46.98 32.86,46.98 32.86,31.74 | 23.96,60.32 23.96,47.62 | C10.- 23.96,60.32 | 35.39,71.75 35.39,65.4 TP4.1 | v54.44,37.46 56.35,37.46

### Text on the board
Top: Top
Bottom: gsi V1.0 Apr 2012 | Bot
